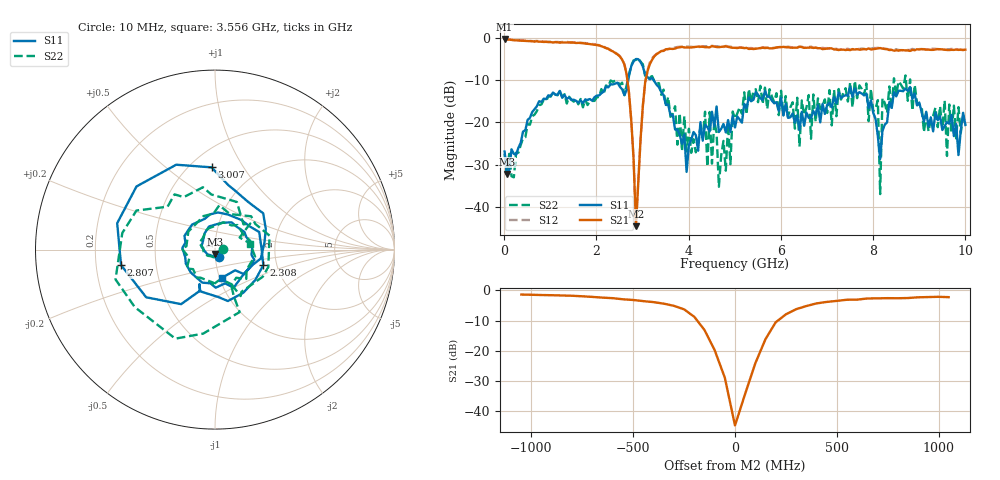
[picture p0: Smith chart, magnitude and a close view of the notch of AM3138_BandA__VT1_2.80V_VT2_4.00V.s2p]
! Date/Time: Tue, Nov 13, 2018 4:42 PM
! Network Analyzer: Agilent Technologies E8364B Rev: A.07.50.67
! Sweep from 0.010 to 10.000 GHz, 201 Points, Sweep Type: LIN
! Power Supply: 2.801 V, 0.000 A
# Hz S DB R 50
!freq MagS11 AngS11 MagS21 AngS21 MagS12 AngS12 MagS22 AngS22
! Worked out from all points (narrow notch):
!   201 points, 10 MHz to 10 GHz, reference 50 ohm
!   highest |S21| = -0.25 dB at 10 MHz (marker M1); lowest = -44.7 dB at 2.857 GHz (marker M2)
!   notch at M2: 42.3 dB deep, 182 MHz wide at half that depth
!   lowest |S11| = -32.2 dB at 59.95 MHz (marker M3), VSWR 1.05, Z = 49.9 - j2.44 ohm
!   |S11| at or under -10 dB: start of sweep to 2.691 GHz; 3.239 GHz to end of sweep
!   |S22| runs from -37.0 to -4.8 dB; largest |S21 - S12| = 0.029
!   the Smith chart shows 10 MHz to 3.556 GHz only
!   S11 on the Smith chart (normalised r, x): 10 MHz: 1.04, -0.08; 2.308 GHz: 1.70, -0.32; 2.807 GHz: 0.31, -0.07; 3.007 GHz: 0.63, +0.73; 3.556 GHz: 1.02, -0.33
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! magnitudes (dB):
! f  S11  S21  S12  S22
! 10 MHz  -26.9  -0.3  -0.3  -27.5
! 59.95 MHz  -32.2  -0.3  -0.3  -32.5
! 1.708 GHz  -15.4  -1.2  -1.2  -16.4
! 2.308 GHz  -11.0  -2.9  -2.8  -10.1
! 2.807 GHz  -5.5  -28.9  -28.8  -5.3
! 2.857 GHz  -5.0  -44.7  -45.0  -5.2
! 3.007 GHz  -6.8  -16.1  -16.1  -6.2
! 3.357 GHz  -11.7  -3.5  -3.5  -10.7
! 3.556 GHz  -15.8  -2.6  -2.7  -14.0
! 3.956 GHz  -31.8  -2.3  -2.0  -26.9
! 4.356 GHz  -20.6  -2.2  -2.0  -17.5
! 4.406 GHz  -21.1  -2.2  -1.9  -30.5
! 4.456 GHz  -22.2  -2.2  -2.0  -17.5
! 4.655 GHz  -22.3  -2.2  -2.0  -35.3
! 5.005 GHz  -21.2  -2.3  -2.2  -19.1
! 6.703 GHz  -17.3  -2.3  -2.3  -13.4
! 7.952 GHz  -14.8  -2.7  -2.5  -12.0
! 8.102 GHz  -23.3  -2.5  -2.3  -14.7
! 8.152 GHz  -28.7  -2.4  -2.4  -37.0
! 8.202 GHz  -22.0  -2.5  -2.4  -14.2
! 8.352 GHz  -15.2  -2.9  -2.7  -11.5
! 10 GHz  -20.6  -2.8  -2.7  -18.9
